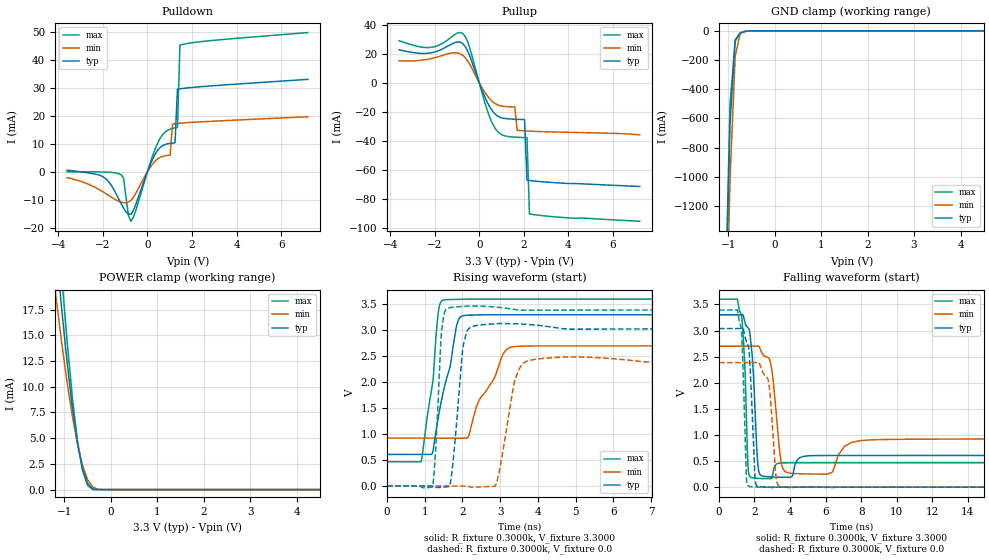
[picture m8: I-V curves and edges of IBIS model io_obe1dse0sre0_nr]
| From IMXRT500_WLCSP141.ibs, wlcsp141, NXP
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[Model] io_obe1dse0sre0_nr
|   Model io_obe1dse0sre0_nr
| Library cells for typ/min/max conditions are connected as defined below:
|  pad - External Pad
|  ipp_do - Core Input
|  ipp_obe - Output Buffer Enable
|  REFH3V3 - vdd1v8
|  REFL3V3 - REFL3V3
|  gnde - gnde
|  ipp_ina235_3v - NC
|  ipp_ina40_3v - NC
|  ipp_ina_mux - NC
|  ipp_ind - NC
|  ipp_ind_1p8v - NC
|  ipp_ind_3v - NC
|  vdd - vdd
|  vdd1v8 - vdd1v8
|  vdda - vdde3v3
|  vdde3v3 - vdde3v3
| All other pins connected to ground
Model_type I/O
Polarity   Non-Inverting
Enable   Active-High
Vinl =   0.9900V
Vinh =   2.3100V
Vmeas =  1.6500V
Cref =   25.0000pF
Rref =   0.5000k
Vref =   0.0V
C_comp   1.8910pF   1.8219pF   2.0892pF
[Temperature Range]   25.0000   0.1250k   -40.0000
[Voltage Range]   3.3000V   2.7000V   3.6000V
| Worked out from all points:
|   slope of the pulldown table from 0 to 0.495 V, typ, clamps not added: 61.4 ohm
|   slope of the pullup table from 0 to 0.495 V, typ, clamps not added: 28.7 ohm
|   GND clamp passes 1 mA (typ) near -0.55 V on its own axis
|   POWER clamp passes 1 mA (typ) near -0.53 V on its own axis
|   rising waveform, R_fixture 0.3000k, V_fixture 3.3000: 20-80 % time 450ps typ, 698ps min, 289ps max; typ from 0.608 V to 3.3 V
|   rising waveform, R_fixture 0.3000k, V_fixture 0.0: 20-80 % time 207ps typ, 322ps min, 135ps max; typ from 0 V to 3.04 V
|   falling waveform, R_fixture 0.3000k, V_fixture 3.3000: 20-80 % time 271ps typ, 331ps min, 214ps max; typ from 3.3 V to 0.608 V
|   falling waveform, R_fixture 0.3000k, V_fixture 0.0: 20-80 % time 232ps typ, 299ps min, 183ps max; typ from 3.04 V to 0 V
[Pulldown]
|Voltage   I(typ)   I(min)   I(max)
-3.6V     580uA      -2.07mA    30uA
-1.95V    -1.94mA    -7.35mA    -60uA
-1.18V    -11.35mA   -10.84mA   -1.013mA
-1.07V    -12.94mA   -11.04mA   -2.193mA
-740mV    -15.14mA   -10.18mA   -17.69mA
360mV     6.495mA    3.971mA    8.469mA
1.02V     10.21mA    5.992mA    15.31mA
1.13V     10.32mA    17.14mA    15.59mA
1.24V     10.39mA    17.26mA    15.78mA
1.35V     29.61mA    17.36mA    15.91mA
1.46V     29.75mA    17.44mA    45.38mA
7.2V      33.13mA    19.73mA    49.89mA
[Pullup]
|Voltage   I(typ)   I(min)   I(max)
-3.6V     22.77mA    15.22mA    29.02mA
-2.15V    20.76mA    16.76mA    24.51mA
-720mV    26.73mA    18.68mA    33.68mA
-500mV    21.29mA    14.62mA    27.43mA
270mV     -10.41mA   -6.963mA   -14.59mA
710mV     -21.5mA    -14.26mA   -31.26mA
1.59V     -25.02mA   -16.58mA   -37.34mA
1.7V      -25.08mA   -32.67mA   -37.43mA
2.03V     -25.25mA   -33.02mA   -37.66mA
2.14V     -66.99mA   -33.11mA   -37.71mA
2.25V     -67.21mA   -33.2mA    -90.22mA
7.2V      -71.34mA   -35.84mA   -95.3mA
[GND_clamp]
|Voltage   I(typ)   I(min)   I(max)
-3.6V     -46.64A    -46.27A    -48.09A
-1.07V    -2.038A    -2.424A    -1.965A
-960mV    -629.9mA   -1.012A    -499.2mA
-850mV    -61.62mA   -174.1mA   -72.03mA
-740mV    -13.6mA    -15.68mA   -16.3mA
-630mV    -2.659mA   -3.244mA   -3.911mA
-410mV    -9.214uA   -49.17uA   -3.123uA
7.2V      0A         0A         0A
[POWER_clamp]
|Voltage   I(typ)   I(min)   I(max)
-3.6V     124.7mA    103.4mA    137.3mA
-1.27V    28.14mA    22.17mA    33.67mA
-1.16V    22.5mA     17.97mA    26.85mA
-1.05V    17.19mA    14.01mA    20.36mA
-940mV    12.34mA    10.39mA    14.37mA
-830mV    8.067mA    7.189mA    9.044mA
-720mV    4.554mA    4.475mA    4.783mA
-610mV    2.051mA    2.374mA    1.895mA
-500mV    596.8uA    974uA      390.7uA
-390mV    63.25uA    246uA      14.24uA
-170mV    55.4nA     1.772uA    16.57nA
7.2V      0A         0A         0A
[Ramp]
| variable   typ   min   max
dV/dt_r  0.7575/0.2239n   0.7280/0.6886n   1.1237/0.1638n
dV/dt_f  0.9021/0.3971n   0.5295/0.4285n   1.3523/0.3390n
R_load = 50.0000
[Rising Waveform]
R_fixture= 0.3000k
V_fixture= 3.3000
V_fixture_min= 2.7000
V_fixture_max= 3.6000
|time   V(typ)   V(min)   V(max)
0s        607.6mV    923.3mV    467.4mV
904.8ps   607.6mV    923.3mV    475.5mV
1.196ns   622.1mV    923.3mV    1.912V
1.402ns   1.495V     923.3mV    3.505V
1.95ns    3.258V     923.4mV    3.6V
2.156ns   3.292V     952.1mV    3.601V
2.42ns    3.296V     1.62V      3.6V
3.138ns   3.3V       2.608V     3.6V
3.858ns   3.3V       2.699V     3.599V
500ns     3.3V       2.7V       3.6V
[Rising Waveform]
R_fixture= 0.3000k
V_fixture= 0.0
V_fixture_min= 0.0
V_fixture_max= 0.0
|time   V(typ)   V(min)   V(max)
0s        91.73nV    1.941uV    241.1nV
1.209ns   -13.15mV   1.921uV    -4.49mV
1.446ns   -25.93mV   1.803uV    2.976V
1.659ns   352uV      1.468uV    3.434V
2.006ns   2.631V     1.441uV    3.46V
2.196ns   3.051V     -17.85mV   3.468V
2.889ns   3.126V     33.07mV    3.449V
3.576ns   3.12V      2.339V     3.388V
4.74ns    3.026V     2.486V     3.389V
500ns     3.038V     2.386V     3.394V
[Falling Waveform]
R_fixture= 0.3000k
V_fixture= 3.3000
V_fixture_min= 2.7000
V_fixture_max= 3.6000
|time   V(typ)   V(min)   V(max)
0s        3.3V       2.7V       3.6V
1.275ns   3.299V     2.7V       3.29V
1.698ns   3.02V      2.7V       228.6mV
2.218ns   352.9mV    2.702V     167.9mV
2.805ns   198.4mV    2.476V     161.8mV
3.61ns    190.4mV    349.6mV    465.2mV
5.861ns   606.5mV    248.2mV    467.4mV
7.451ns   607.4mV    855.2mV    467.4mV
11.47ns   607.7mV    920mV      467.4mV
500ns     607.6mV    923.3mV    467.4mV
[Falling Waveform]
R_fixture= 0.3000k
V_fixture= 0.0
V_fixture_min= 0.0
V_fixture_max= 0.0
|time   V(typ)   V(min)   V(max)
0s        3.038V     2.386V     3.394V
1.25ns    3.038V     2.386V     3.059V
1.592ns   2.757V     2.386V     52.93mV
1.728ns   2.471V     2.386V     13.41mV
2.06ns    94.28mV    2.385V     3.842mV
2.766ns   3.069mV    2.065V     -3.183mV
2.95ns    2.378mV    1.482V     -12.94mV
3.331ns   1.642mV    42.43mV    829.5uV
6.327ns   267uV      -8.066mV   13.14uV
500ns     1.148uV    3.187uV    858.6nV
